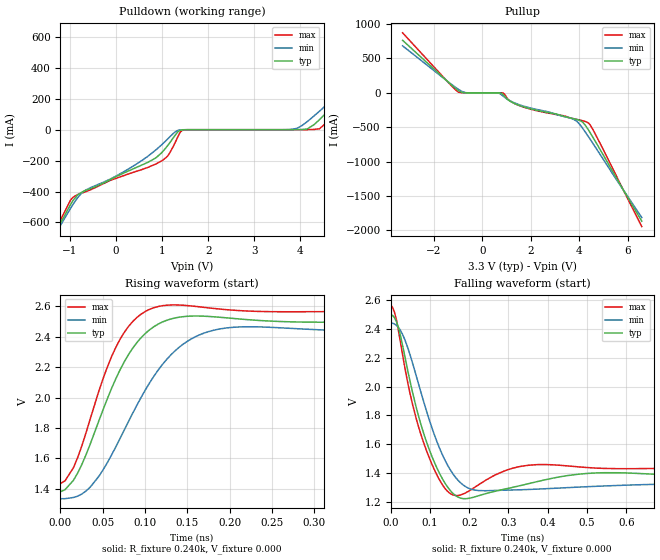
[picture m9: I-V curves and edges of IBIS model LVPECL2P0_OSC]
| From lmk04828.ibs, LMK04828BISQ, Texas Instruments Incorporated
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[Model]   LVPECL2P0_OSC
Model_type   Output
Polarity   Non-Inverting
Vmeas = 1.99
Vref = 1.99
Cref = 0pF
Rref = 240
|   typ   min   max
|   (nom PVT)   (fast PVT)   (slow PVT)
C_comp   0.2109p   0.1807p   0.2310p
|C_comp (Low state)   0.2109p   0.1807p   0.2310p
|C_comp (High state)   0.9933p   0.9197p   1.0724p
[Voltage Range]   3.3   3.15   3.45
[Temperature Range]   27   125   -40
[Pullup Reference]   3.3   3.15   3.45
[Pulldown Reference]   0   0   0
[Power Clamp Reference]   3.3   3.15   3.45
[GND Clamp Reference]   0   0   0
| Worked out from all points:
|   slope of the pulldown table from 0 to 0.495 V, typ, clamps not added: 7.42 ohm
|   falling waveform, R_fixture 0.240k, V_fixture 0.000: 20-80 % time 61.8ps typ, 77.5ps min, 55.1ps max; typ from 2.5 V to 1.38 V
|   rising waveform, R_fixture 0.240k, V_fixture 0.000: 20-80 % time 50.8ps typ, 66.8ps min, 42.4ps max; typ from 1.38 V to 2.5 V
[Pulldown]
|   Voltage   I(typ)   I(min)   I(max)
-3.3V     -1.869A    -1.737A    -2.051A
-1.28V    -652.5mA   -661.4mA   -639.7mA
-983.4mV  -485.5mA   -510mA     -456.6mA
-825mV    -421.3mA   -438.6mA   -419mA
986.7mV   -150.5mA   -99.33mA   -202.4mA
1.145V    -93.97mA   -53.27mA   -161.1mA
1.452V    -583uA     -287.8uA   -1.99mA
3.769V    8.124uA    1.31mA     128.1nA
4.155V    6.485mA    54.36mA    475.7uA
4.412V    65.2mA     120mA      6.277mA
5.145V    293.7mA    319.5mA    257.9mA
6.59V     761.2mA    723.2mA    811.3mA
[Pullup]
|   Voltage   I(typ)   I(min)   I(max)
-3.3V     764.4mA    683.9mA    873mA
-983.4mV  30.09mA    49.29mA    9.236mA
-686.4mV  508.5uA    3.353mA    377.6uA
561mV     -3.193uA   -260.9uA   -15.17nA
848.1mV   -23.41mA   -44.36mA   -1.6mA
1.115V    -113.3mA   -109.9mA   -110.4mA
1.531V    -182.7mA   -172.8mA   -185.6mA
3.739V    -372.4mA   -379.6mA   -372.9mA
4.125V    -420.2mA   -504.9mA   -403.5mA
4.392V    -543.2mA   -640.9mA   -440.5mA
4.966V    -883.9mA   -948.6mA   -801.6mA
6.59V     -1.865A    -1.813A    -1.943A
[Ramp]
R_load = 240
|   typ   min   max
dV/dt_r   0.669407/5.08194e-11   0.660633/6.67586e-11   0.676564/4.24188e-11
dV/dt_f   0.66946/6.18152e-11   0.660583/7.75013e-11   0.676594/5.50565e-11
[Falling Waveform]
R_fixture = 0.240k
V_fixture = 0.000
V_fixture_min = 0.000
V_fixture_max = 0.000
C_fixture = 0.000
|  time   V(typ)   V(min)   V(max)
0s        2.496V     2.437V     2.565V
14.91ps   2.449V     2.424V     2.46V
34.91ps   2.226V     2.333V     2.151V
79.91ps   1.713V     1.935V     1.645V
124.9ps   1.397V     1.571V     1.352V
159.9ps   1.258V     1.391V     1.249V
214.9ps   1.237V     1.284V     1.304V
369.9ps   1.34V      1.29V      1.46V
544.9ps   1.404V     1.312V     1.434V
1.87ns    1.38V      1.336V     1.435V
[Rising Waveform]
R_fixture = 0.240k
V_fixture = 0.000
V_fixture_min = 0.000
V_fixture_max = 0.000
C_fixture = 0.000
|  time   V(typ)   V(min)   V(max)
0s        1.381V     1.336V     1.435V
15.37ps   1.456V     1.343V     1.539V
35.37ps   1.697V     1.413V     1.863V
55.37ps   1.992V     1.572V     2.2V
70.37ps   2.182V     1.731V     2.382V
95.37ps   2.394V     2.002V     2.548V
125.4ps   2.507V     2.25V      2.606V
165.4ps   2.535V     2.414V     2.595V
215.4ps   2.514V     2.464V     2.57V
1.885ns   2.496V     2.437V     2.565V
